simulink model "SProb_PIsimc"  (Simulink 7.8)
settings: Solver=ode3  StartTime=0.0  StopTime=50  FixedStep=0.01  RelTol=1e-6
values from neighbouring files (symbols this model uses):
  delay = delayv(i)    [example.m]    (also in IAE_Simulink.m; Robustness_SP.m; Robustness_SP_P.m; Robustness_SP_PI.m)
libraries: simulink x2

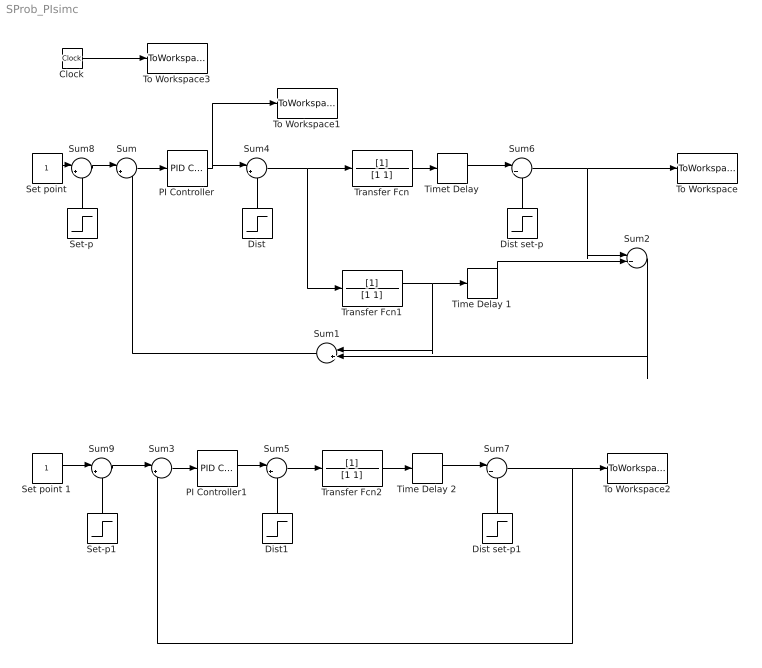
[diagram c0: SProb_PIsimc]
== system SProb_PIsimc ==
  Clock : Clock
  Dist : Step  Time=0  After=0  SampleTime=0
  Dist set-p : Step  Time=20  After=0  SampleTime=0
  Dist set-p1 : Step  Time=20  After=0  SampleTime=0
  Dist1 : Step  Time=0  After=0  SampleTime=0
  PI Controller : simulink/Continuous/PID Controller  Controller=PI  TimeDomain=Continuous-time  SampleTime=1  IntegratorMethod=Forward Euler  FilterMethod=Forward Euler  Form=Ideal  P=3  I=1  D=0  N=100  InitialConditionSource=internal  InitialConditionForIntegrator=0  InitialConditionForFilter=0  ExternalReset=none  LimitOutput=off  UpperSaturationLimit=inf  LowerSaturationLimit=-inf  LinearizeAsGain=off  AntiWindupMode=none  Kb=1  TrackingMode=off  Kt=1  PParamMin=[]  PParamMax=[]  IParamMin=[]  IParamMax=[]  DParamMin=[]  DParamMax=[]  NParamMin=[]  NParamMax=[]  KbParamMin=[]  KbParamMax=[]  KtParamMin=[]  KtParamMax=[]  POutMin=[]  POutMax=[]  IOutMin=[]  IOutMax=[]  DOutMin=[]  DOutMax=[]  NOutMin=[]  NOutMax=[]  KbOutMin=[]  KbOutMax=[]  KtOutMin=[]  KtOutMax=[]  IntegratorOutMin=[]  IntegratorOutMax=[]  FilterOutMin=[]  FilterOutMax=[]  SumOutMin=[]  SumOutMax=[]  SumI1OutMin=[]  SumI1OutMax=[]  SumI2OutMin=[]  SumI2OutMax=[]  SumI3OutMin=[]  SumI3OutMax=[]  SumDOutMin=[]  SumDOutMax=[]  SaturationOutMin=[]  SaturationOutMax=[]  IntegratorContinuousStateAttributes=''  IntegratorStateMustResolveToSignalObject=off  IntegratorRTWStateStorageClass=Auto  FilterContinuousStateAttributes=''  FilterStateMustResolveToSignalObject=off  FilterRTWStateStorageClass=Auto
  PI Controller1 : simulink/Continuous/PID Controller  Controller=PI  TimeDomain=Continuous-time  SampleTime=1  IntegratorMethod=Forward Euler  FilterMethod=Forward Euler  Form=Ideal  P=0.5  I=1  D=0  N=100  InitialConditionSource=internal  InitialConditionForIntegrator=0  InitialConditionForFilter=0  ExternalReset=none  LimitOutput=off  UpperSaturationLimit=inf  LowerSaturationLimit=-inf  LinearizeAsGain=off  AntiWindupMode=none  Kb=1  TrackingMode=off  Kt=1  PParamMin=[]  PParamMax=[]  IParamMin=[]  IParamMax=[]  DParamMin=[]  DParamMax=[]  NParamMin=[]  NParamMax=[]  KbParamMin=[]  KbParamMax=[]  KtParamMin=[]  KtParamMax=[]  POutMin=[]  POutMax=[]  IOutMin=[]  IOutMax=[]  DOutMin=[]  DOutMax=[]  NOutMin=[]  NOutMax=[]  KbOutMin=[]  KbOutMax=[]  KtOutMin=[]  KtOutMax=[]  IntegratorOutMin=[]  IntegratorOutMax=[]  FilterOutMin=[]  FilterOutMax=[]  SumOutMin=[]  SumOutMax=[]  SumI1OutMin=[]  SumI1OutMax=[]  SumI2OutMin=[]  SumI2OutMax=[]  SumI3OutMin=[]  SumI3OutMax=[]  SumDOutMin=[]  SumDOutMax=[]  SaturationOutMin=[]  SaturationOutMax=[]  IntegratorContinuousStateAttributes=''  IntegratorStateMustResolveToSignalObject=off  IntegratorRTWStateStorageClass=Auto  FilterContinuousStateAttributes=''  FilterStateMustResolveToSignalObject=off  FilterRTWStateStorageClass=Auto
  Set point : Constant
  Set point 1 : Constant
  Set-p : Step  Time=10  SampleTime=0
  Set-p1 : Step  Time=10  SampleTime=0
  Sum : Sum  Inputs=|+-
  Sum{1,4..9} (7 alike) : Sum  Inputs=|++
  Sum2 : Sum  Inputs=|+-
  Sum3 : Sum  Inputs=|+-
  Time Delay 1 : TransportDelay
  Time Delay 2 : TransportDelay  DelayTime=delay
  Timet Delay : TransportDelay  DelayTime=delay
  To Workspace : ToWorkspace  VariableName=Ysp  SampleTime=-1  SaveFormat=Array
  To Workspace1 : ToWorkspace  VariableName=usp  SampleTime=-1  SaveFormat=Structure
  To Workspace2 : ToWorkspace  VariableName=Ypi  SampleTime=-1  SaveFormat=Array
  To Workspace3 : ToWorkspace  VariableName=time  SampleTime=-1  SaveFormat=Array
  Transfer Fcn : TransferFcn  Denominator=[1 1]
  Transfer Fcn1 : TransferFcn  Denominator=[1 1]
  Transfer Fcn2 : TransferFcn  Denominator=[1 1]
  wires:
  Sum/1 -> PI Controller/1
  PI Controller/1 -> To Workspace1/1, Sum4/1
  Transfer Fcn/1 -> Timet Delay/1
  Time Delay 1/1 -> Sum2/2
  Sum2/1 -> Sum1/2
  Sum1/1 -> Sum/2
  Transfer Fcn2/1 -> Time Delay 2/1
  Sum3/1 -> PI Controller1/1
  Clock/1 -> To Workspace3/1
  Sum4/1 -> Transfer Fcn/1, Transfer Fcn1/1
  PI Controller1/1 -> Sum5/1
  Dist1/1 -> Sum5/2
  Sum5/1 -> Transfer Fcn2/1
  Timet Delay/1 -> Sum6/1
  Dist set-p/1 -> Sum6/2
  Sum6/1 -> Sum2/1, To Workspace/1
  Time Delay 2/1 -> Sum7/1
  Dist set-p1/1 -> Sum7/2
  Sum7/1 -> Sum3/2, To Workspace2/1
  Dist/1 -> Sum4/2
  Set point/1 -> Sum8/1
  Sum8/1 -> Sum/1
  Set-p/1 -> Sum8/2
  Set point 1/1 -> Sum9/1
  Sum9/1 -> Sum3/1
  Set-p1/1 -> Sum9/2
  Transfer Fcn1/1 -> Time Delay 1/1, Sum1/1
